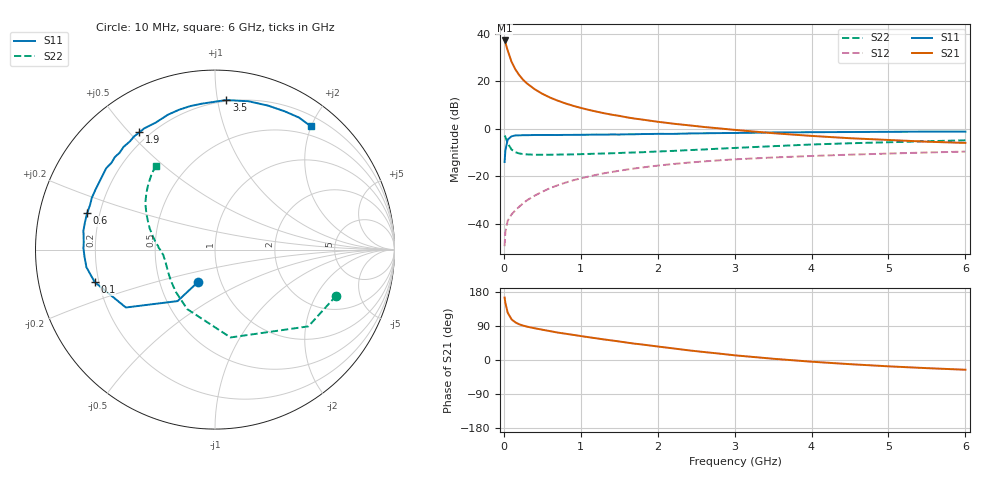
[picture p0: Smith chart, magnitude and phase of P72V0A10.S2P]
! SIEMENS Small Signal Semiconductors
! BFP196
! Si NPN RF Bipolar Junction Transistor in SOT143
! VCE = 2 V  IC = 100 mA
! Common Emitter S-Parameters:  May  1996
# GHz  S  MA  R  50
!  f  S11  S21  S12  S22
! GHz  MAG  ANG  MAG  ANG  MAG  ANG  MAG  ANG
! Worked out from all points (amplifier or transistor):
!   36 points, 10 MHz to 6 GHz, reference 50 ohm
!   highest |S21| = 37.1 dB at 10 MHz (marker M1)
!   |S21| within 3 dB of that: start of sweep to 38.96 MHz
!   unconditionally stable (mu >= 1): 261 MHz to end of sweep
!   at 250 MHz: K = 0.99, MSG = 26.0 dB, |S12| = -31.3 dB
!   at 1.4 GHz: K = 1.11, MAG = 10.0 dB, |S12| = -18.2 dB
!   at 6 GHz: K = 1.02, MAG = 1.0 dB, |S12| = -9.6 dB
!   S11 on the Smith chart (normalised r, x): 10 MHz: 0.78, -0.29; 100 MHz: 0.18, -0.13; 600 MHz: 0.15, +0.14; 1.9 GHz: 0.16, +0.53; 3.5 GHz: 0.19, +1.06; 6 GHz: 0.35, +2.00
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0.01  0.2002 -117.4  71.99 164.8  0.0034 70.9  0.7227 -20.8
0.02  0.3547 -126.0  64.97 150.6  0.0068 66.8  0.6736 -39.4
0.05  0.5922 -147.0  44.25 125.0  0.0116 50.7  0.497 -80.0
0.1  0.6943 -164.9  25.67 107.3  0.0158 50.8  0.366 -115.0
0.15  0.7231 -172.2  17.72 99.2  0.0193 55.3  0.3215 -132.6
0.2  0.7281 -176.9  13.46 94.2  0.023 59.4  0.303 -143.0
0.25  0.733 179.4  10.74 90.8  0.0271 61.5  0.2935 -150.4
0.3  0.7324 176.8  8.999 88.1  0.0313 64.6  0.2894 -154.8
0.4  0.7406 171.8  6.805 83.8  0.0392 66.4  0.285 -161.3
0.5  0.7405 168.1  5.443 80.0  0.0475 67.5  0.2842 -165.4
0.6  0.7409 164.1  4.538 76.2  0.0564 67.4  0.2848 -168.3
0.7  0.7392 160.3  3.902 72.4  0.0649 67.0  0.2865 -170.4
0.8  0.7445 157.2  3.419 69.4  0.0736 65.7  0.2883 -172.2
1.1  0.75 146.7  2.505 60.2  0.099 62.5  0.2959 -176.4
1.4  0.7597 137.2  1.982 51.7  0.1231 58.2  0.3054 -179.8
1.9  0.7771 122.8  1.48 38.2  0.1609 50.3  0.3275 174.5
2.2  0.7809 115.0  1.282 30.6  0.1816 45.6  0.3427 170.6
2.8  0.8113 99.8  1.019 16.9  0.2171 36.2  0.3824 162.1
3.5  0.8357 85.7  0.808 3.3  0.2491 25.9  0.4308 152.5
4.5  0.8549 69.8  0.633 -11.0  0.2856 13.7  0.4961 140.4
5.5  0.8718 57.6  0.535 -21.5  0.3173 2.8  0.5474 130.3
6  0.8703 52.1  0.504 -25.7  0.3316 -3.0  0.5718 125.3
